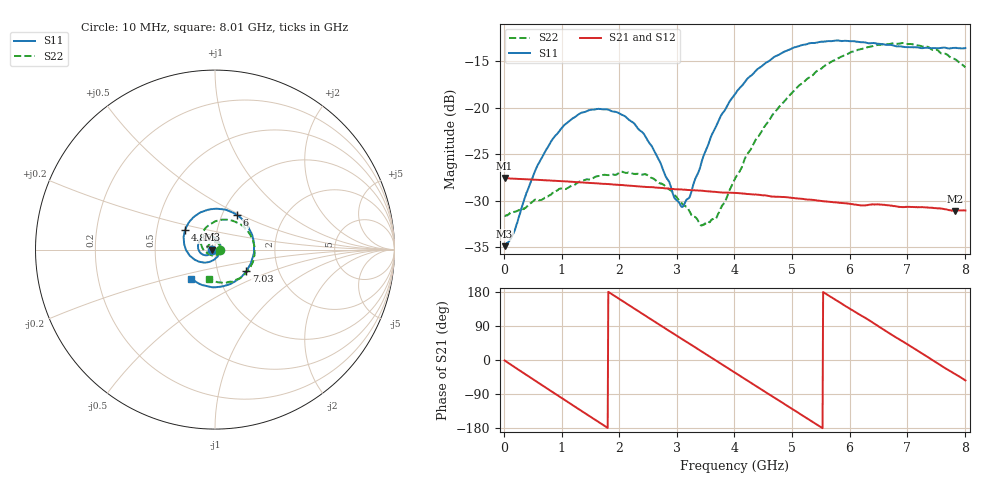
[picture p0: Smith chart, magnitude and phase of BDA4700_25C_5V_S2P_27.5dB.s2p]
!Agilent Technologies,E5071B,MY42404982,A.09.10
!Date: Mon Oct 20 13:40:22 2025
!Data & Calibration Information:
!Freq	S11:SOLT2(ON)	S21:SOLT2(ON)	S12:SOLT2(ON)	S22:SOLT2(ON)
# Hz S RI R 50
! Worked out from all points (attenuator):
!   801 points, 10 MHz to 8.01 GHz, reference 50 ohm
!   highest |S21| = -27.57 dB at 10 MHz (marker M1); lowest = -31.1 dB at 7.83 GHz (marker M2)
!   lowest |S11| = -34.9 dB at 10 MHz (marker M3), VSWR 1.04, Z = 48.2 - j0.0956 ohm
!   |S11| at or under -10 dB: start of sweep to end of sweep
!   |S22| runs from -32.7 to -13.0 dB; largest |S21 - S12| = 0.00035
!   S11 on the Smith chart (normalised r, x): 10 MHz: 0.96, -0.00; 4.85 GHz: 0.70, +0.16; 6 GHz: 1.18, +0.48; 7.03 GHz: 1.37, -0.34; 8.01 GHz: 0.73, -0.25
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1e7  -0.018 -0.000991  0.0418 -0.000898  0.0418 -0.000949  0.0262 -0.000843
1.6e8  -0.0188 -0.00937  0.0398 -0.0117  0.0398 -0.0118  0.0264 -0.00754
5.4e8  -0.0356 -0.0288  0.0237 -0.0333  0.0237 -0.0334  0.0157 -0.0278
7.7e8  -0.0536 -0.0315  0.00887 -0.0396  0.00886 -0.0397  0.00107 -0.0335
1.35e9  -0.094 0.00448  -0.028 -0.0281  -0.028 -0.028  -0.036 -0.0178
2.09e9  -0.052 0.0737  -0.0338 0.0178  -0.0339 0.0178  -0.0292 0.034
2.42e9  -0.00982 0.072  -0.0188 0.0324  -0.0189 0.0325  -0.00499 0.0434
2.68e9  0.0175 0.0502  -0.00316 0.0369  -0.00318 0.037  0.0128 0.0374
2.96e9  0.0299 0.0128  0.0137 0.0337  0.0137 0.0337  0.0254 0.0226
3.11e9  0.0279 -0.00938  0.0216 0.0291  0.0216 0.0291  0.028 0.0106
3.42e9  0.00219 -0.0498  0.0328 0.0143  0.0328 0.0143  0.0197 -0.0123
3.54e9  -0.0138 -0.0611  0.0347 0.00736  0.0348 0.00729  0.0129 -0.0202
3.7e9  -0.0416 -0.0702  0.0351 -0.00206  0.0351 -0.00216  -0.000645 -0.0261
4.01e9  -0.1003 -0.0623  0.0291 -0.019  0.0291 -0.019  -0.0322 -0.0258
4.85e9  -0.1667 0.1088  -0.0136 -0.0301  -0.0135 -0.0302  -0.0757 0.0752
5.35e9  -0.0733 0.2103  -0.0304 -0.00949  -0.0305 -0.0096  -0.0154 0.1478
6e9  0.1231 0.1918  -0.0217 0.0213  -0.0218 0.0213  0.1312 0.1473
6.68e9  0.2176 -0.00693  0.0095 0.0283  0.00952 0.0282  0.2198 0.000287
7.03e9  0.1745 -0.1198  0.0228 0.0184  0.0228 0.0183  0.1989 -0.0936
7.46e9  0.0503 -0.203  0.0288 -0.00113  0.0289 -0.00117  0.1106 -0.1726
7.83e9  -0.0784 -0.1945  0.0223 -0.0167  0.0224 -0.0168  0.0132 -0.1817
8.01e9  -0.1324 -0.1621  0.0165 -0.0226  0.0165 -0.0226  -0.0307 -0.162
